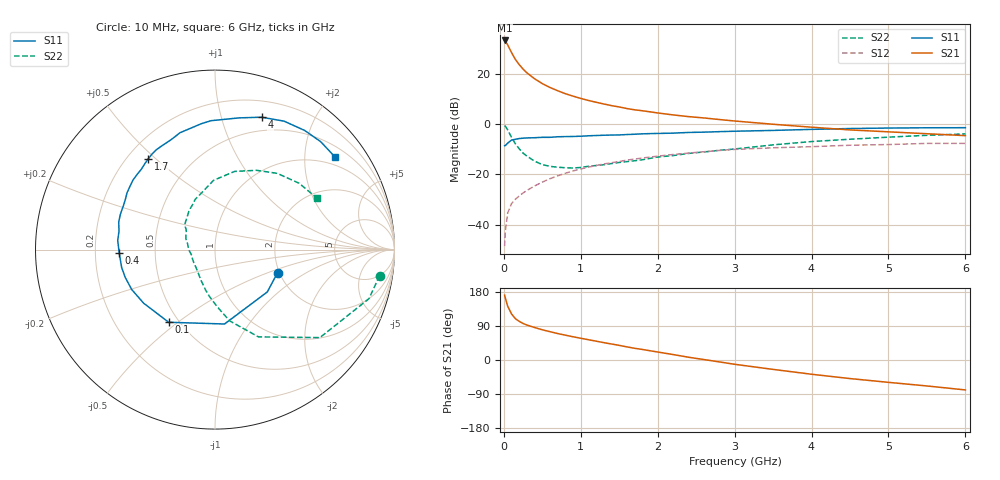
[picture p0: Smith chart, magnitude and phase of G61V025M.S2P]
! SIEMENS Small Signal Semiconductors
! BFG193
! Si NPN RF Bipolar Junction Transistor in SOT223
! VCE = 1 V  IC = 25 mA
! Common Emitter S-Parameters:  August  1996
# GHz  S  MA  R  50
!  f  S11  S21  S12  S22
! GHz  MAG  ANG  MAG  ANG  MAG  ANG  MAG  ANG
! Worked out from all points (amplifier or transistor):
!   36 points, 10 MHz to 6 GHz, reference 50 ohm
!   highest |S21| = 33.1 dB at 10 MHz (marker M1)
!   |S21| within 3 dB of that: start of sweep to 70.47 MHz
!   unconditionally stable (mu >= 1): 511 MHz to 2.968 GHz; 3.196 GHz to 3.557 GHz
!   at 250 MHz: K = 0.82, MSG = 24.5 dB, |S12| = -27.3 dB
!   at 1.4 GHz: K = 1.07, MAG = 9.7 dB, |S12| = -15.4 dB
!   at 6 GHz: K = 0.97, MSG = 1.5 dB, |S12| = -7.7 dB
!   S11 on the Smith chart (normalised r, x): 10 MHz: 1.95, -0.58; 100 MHz: 0.44, -0.46; 400 MHz: 0.30, -0.02; 1.7 GHz: 0.28, +0.47; 4 GHz: 0.36, +1.35; 6 GHz: 0.76, +2.75
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0.01  0.3716 -20.3  45.14 171.1  0.0038 86.3  0.9286 -9.0
0.02  0.3749 -39.0  43.89 163.2  0.0076 79.8  0.9002 -17.7
0.05  0.4179 -82.7  36.85 141.9  0.0172 65.3  0.7629 -40.0
0.1  0.4801 -122.5  26.01 121.6  0.0265 57.2  0.5434 -63.5
0.15  0.4972 -143.1  19.01 109.1  0.0323 54.2  0.4053 -78.4
0.2  0.5146 -154.4  15 102.0  0.0375 55.9  0.3219 -87.3
0.25  0.5234 -162.7  12.2 96.4  0.043 56.5  0.265 -96.4
0.3  0.5296 -169.1  10.31 92.2  0.0482 58.2  0.2309 -103.2
0.4  0.534 -177.9  7.849 85.7  0.0593 58.9  0.1834 -116.2
0.5  0.5445 174.5  6.31 79.7  0.0705 59.5  0.157 -127.5
0.6  0.5444 169.3  5.288 74.7  0.0825 58.8  0.1448 -137.3
0.7  0.5582 163.9  4.555 69.8  0.0939 58.0  0.1392 -147.2
0.9  0.5658 154.5  3.558 61.3  0.1176 54.7  0.1338 -165.5
1.1  0.5835 147.1  2.924 53.5  0.1395 51.5  0.1452 -178.7
1.7  0.6269 126.6  1.91 30.9  0.202 38.7  0.1869 148.7
2.2  0.659 111.9  1.513 14.4  0.2488 26.5  0.2367 131.5
2.8  0.7052 96.3  1.226 -5.0  0.2991 12.2  0.3008 111.5
3.5  0.7455 79.8  0.988 -24.8  0.3377 -5.5  0.3859 91.2
4  0.7821 70.6  0.864 -37.6  0.3554 -15.1  0.4488 76.0
4.5  0.8126 61.7  0.763 -49.0  0.3794 -24.9  0.499 62.3
5.5  0.8416 45.6  0.641 -68.5  0.4126 -47.1  0.5967 38.3
6  0.8447 37.6  0.588 -79.0  0.4128 -59.8  0.6364 26.8
